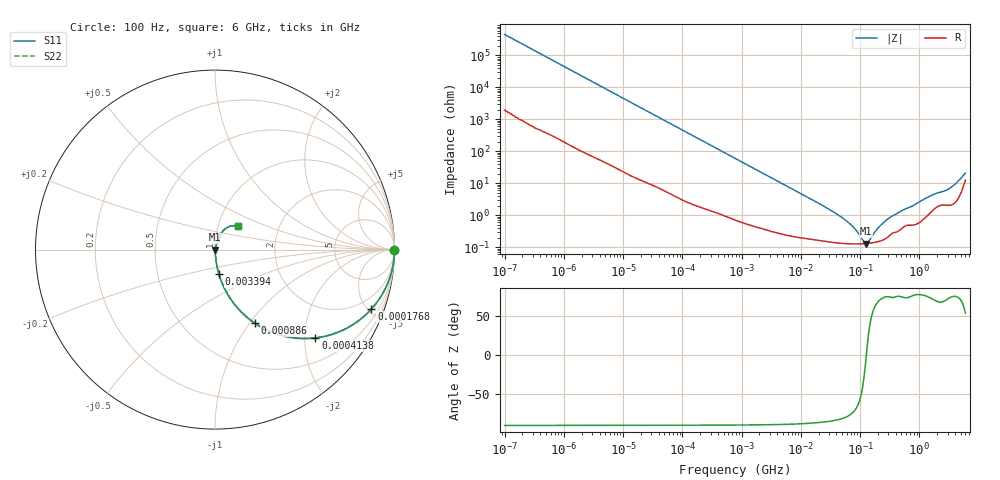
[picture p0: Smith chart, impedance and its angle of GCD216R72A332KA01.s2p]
!Murata Part Number: GCD216R72A332KA01
!These Parameters are Measured in Series Mode Connection
!Data Generated on Jan 08, 2026
!  o--ll--o
!Port1  Port2
!  o------o
!Operation Temp=25[degC], DC Bias Voltage=0[V]
!Freq. Start=100[Hz] Stop=6[GHz] 401[Steps]
# Hz S RI R 50
!Freq.(Hz) S11(Real) S11(Imag) S21(Real) S21(Imag) S12(Real) S12(Imag) S22(Real) S22(Imag)
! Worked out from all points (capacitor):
!   401 points, 100 Hz to 6 GHz, reference 50 ohm
!   read as one part in series: C = 3.5 nF near 109 Hz
!   lowest |Z| = 130 mohm at 127.6 MHz (marker M1)
!   series resonance near 127.7 MHz, so ESL is about 440 pH
!   S11 on the Smith chart (normalised r, x): 100 Hz: open; 176.8 kHz: 1.04, -5.26; 413.8 kHz: 1.02, -2.26; 886 kHz: 1.01, -1.06; 3.394 MHz: 1.01, -0.28; 6 GHz: 1.25, +0.33
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100  1 -0.00022  1e-06 0.00022  1e-06 0.00022  1 -0.00022
2008  1 -0.00439  3.82e-05 0.00439  3.82e-05 0.00439  1 -0.00439
40335  0.9919 -0.0865  0.00808 0.0865  0.00808 0.0865  0.9919 -0.0865
98762  0.9554 -0.2031  0.0446 0.2031  0.0446 0.2031  0.9554 -0.2031
176758  0.8718 -0.3307  0.1282 0.3307  0.1282 0.3307  0.8718 -0.3307
413847  0.5592 -0.4915  0.4408 0.4915  0.4408 0.4915  0.5592 -0.4915
774597  0.2702 -0.4382  0.7298 0.4382  0.7298 0.4382  0.2702 -0.4382
885955  0.2216 -0.4092  0.7784 0.4092  0.7784 0.4092  0.2216 -0.4092
1585629  0.0844 -0.2704  0.9156 0.2704  0.9156 0.2704  0.0844 -0.2704
3394479  0.0219 -0.1359  0.9781 0.1359  0.9781 0.1359  0.0219 -0.1359
1.555665e7  0.00266 -0.0303  0.9973 0.0303  0.9973 0.0303  0.00266 -0.0303
5.699437e7  0.00134 -0.00687  0.9987 0.00687  0.9987 0.00687  0.00134 -0.00687
7.797396e7  0.00128 -0.00394  0.9987 0.00394  0.9987 0.00394  0.00128 -0.00394
1.166697e8  0.00129 -0.000699  0.9987 0.000699  0.9987 0.000699  0.00129 -0.000699
1.275994e8  0.0013 -8.3e-06  0.9987 8.3e-06  0.9987 8.3e-06  0.0013 -8.3e-06
1.395531e8  0.00132 0.000683  0.9987 -0.000683  0.9987 -0.000683  0.00132 0.000683
2.088084e8  0.00153 0.00398  0.9985 -0.00398  0.9985 -0.00398  0.00153 0.00398
3.124326e8  0.00234 0.00796  0.9977 -0.00796  0.9977 -0.00796  0.00234 0.00796
1.497423e9  0.0127 0.0369  0.9873 -0.0369  0.9873 -0.0369  0.0127 0.0369
3.065283e9  0.0236 0.0592  0.9764 -0.0592  0.9764 -0.0592  0.0236 0.0592
4.586474e9  0.0449 0.1048  0.9551 -0.1048  0.9551 -0.1048  0.0449 0.1048
6e9  0.1302 0.1294  0.8698 -0.1294  0.8698 -0.1294  0.1302 0.1294
